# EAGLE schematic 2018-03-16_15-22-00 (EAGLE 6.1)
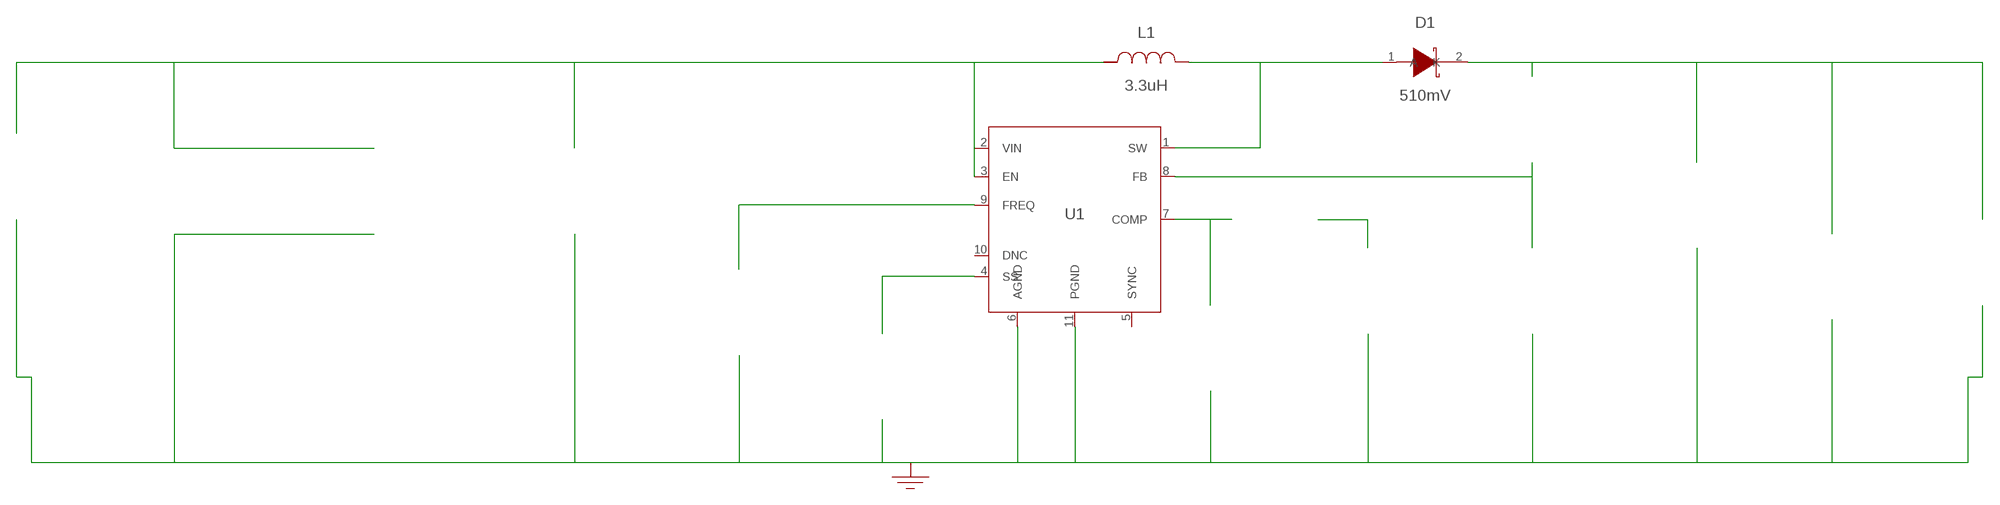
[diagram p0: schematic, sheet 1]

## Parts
CCOMP  100nF  08053C104JAZ2A08053C104JAZ2A  [0805]  (not placed on a sheet)
CCOMP2  10nF  GCM2195C1H103JA16DGCM2195C1H103JA16D  [0805]  (not placed on a sheet)
CIN  10uF  GRM219R61A106KE44DGRM219R61A106KE44D  [0805]  (not placed on a sheet)
CIN_2  10uF  GRM219R61A106KE44DGRM219R61A106KE44D  [0805]  (not placed on a sheet)
CIN_3  10uF  GRM219R61A106KE44DGRM219R61A106KE44D  [0805]  (not placed on a sheet)
CINX  100nF  CC0805KRX7R8BB104CC0805KRX7R8BB104  [0805]  (not placed on a sheet)
COUT  22uF  GRM32ER61C226ME20LGRM32ER61C226ME20L  [1210]  (not placed on a sheet)
COUTX  1uF  EMK107B7105KA-TEMK107B7105KA-T  [0603]  (not placed on a sheet)
CSS  22nF  GRM033R60J223KE01DGRM033R60J223KE01D  [0201]  (not placed on a sheet)
D1  510mV  MBRD835LT4GMBRD835LT4G  [DPAK]
GND  WB_GND  WB_GNDWB_GND  [WB_GND]
IOUT  WB_CURRENT_LOAD  WB_CURRENT_LOADWB_CURRENT_LOAD  [WB_CURRENT_LOAD]  (not placed on a sheet)
L1  3.3uH  XAL5030-332MEBXAL5030-332MEB  [XAL5030]
RCOMP  953  CRCW0402953RFKEDCRCW0402953RFKED  [0402]  (not placed on a sheet)
RFBB  10k  RR1220P-103-DRR1220P-103-D  [0805]  (not placed on a sheet)
RFBT  86.6k  CRCW040286K6FKEDCRCW040286K6FKED  [0402]  (not placed on a sheet)
RT  60.4k  CRCW040260K4FKEDCRCW040260K4FKED  [0402]  (not placed on a sheet)
U1  TPS55340RTER  TPS55340RTERTPS55340RTER  [S-PWQFN-N16]
VIN  WB_BATTERY  WB_BATTERYWB_BATTERY  [WB_BATTERY]  (not placed on a sheet)

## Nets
0: Ccomp2.1@1 Ccomp.2@2 Cin.2@2 Cin_2.2@2 Cin_3.2@2 Cinx.2@2 Cout.2@2 Coutx.2@2 Css.2@2 GND.1 Iout.-@2 Rfbb.2@2 Rt.2@2 U1.6(AGND) U1.11(PGND) U1.12(PGND) U1.13(PGND) U1.17(ETPAD) Vin.-@2
1: Cin.1@1 Cin_2.1@1 Cin_3.1@1 Cinx.1@1 L1.2 U1.2(VIN) U1.3(EN) Vin.+@1
2: Rt.1@1 U1.9(FREQ)
3: Css.1@1 U1.4(SS)
4: Ccomp2.2@2 Rcomp.2@2 U1.7(COMP)
5: D1.1(A) D1.3(A) L1.1 U1.1(SW) U1.15(SW) U1.16(SW)
6: Ccomp.1@1 Rcomp.1@1
7: Rfbb.1@1 Rfbt.2@2 U1.8(FB)
8: Cout.1@1 Coutx.1@1 D1.2(K) Iout.+@1 Rfbt.1@1
Unconnected: CCOMP2.1 CCOMP2.2 CCOMP.1 CCOMP.2 CIN.1 CIN.2 CIN_2.1 CIN_2.2 CIN_3.1 CIN_3.2 CINX.1 CINX.2 COUT.1 COUT.2 COUTX.1 COUTX.2 CSS.1 CSS.2 IOUT.1(+) IOUT.2(-) RCOMP.1 RCOMP.2 RFBB.1 RFBB.2 RFBT.1 RFBT.2 RT.1 RT.2 U1.5(SYNC) U1.10(DNC) U1.14(DNC) VIN.1(+) VIN.2(-)

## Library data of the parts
CCOMP = AcceleratedDesigns_Lib:08053C104JAZ2A; Cap: 1.0E-7; Datasheet_URL: http://catalogs.avx.com/SurfaceMount.pdf; ESR: 0.0; IRMS: 0.0; Manufacturer_Name: AVX; Manufacturer_Part_Number: 08053C104JAZ2A; VDC: 25.0; Vendor: AVX
CCOMP2 = AcceleratedDesigns_Lib:GCM2195C1H103JA16D; Cap: 1.0E-8; Datasheet_URL: http://www.murata.com/products/catalog/pdf/c03e.pdf; ESR: 0.0; IRMS: 0.0; Manufacturer_Name: MuRata; Manufacturer_Part_Number: GCM2195C1H103JA16D; VDC: 50.0; Vendor: MuRata
CIN CIN_2 CIN_3 = AcceleratedDesigns_Lib:GRM219R61A106KE44D; Cap: 1.0E-5; ESR: 0.0050; IRMS: 0.0; Manufacturer_Name: MuRata; Manufacturer_Part_Number: GRM219R61A106KE44D; VDC: 10.0; Vendor: MuRata
CINX = AcceleratedDesigns_Lib:CC0805KRX7R8BB104; Cap: 1.0E-7; ESR: 0.0; IRMS: 0.0; Manufacturer_Name: Yageo America; Manufacturer_Part_Number: CC0805KRX7R8BB104; VDC: 25.0; Vendor: Yageo America
COUT = AcceleratedDesigns_Lib:GRM32ER61C226ME20L; Cap: 2.2E-5; ESR: 0.0020; IRMS: 0.0; Manufacturer_Name: MuRata; Manufacturer_Part_Number: GRM32ER61C226ME20L; VDC: 16.0; Vendor: MuRata
COUTX = AcceleratedDesigns_Lib:EMK107B7105KA-T; Cap: 1.0E-6; ESR: 0.0; IRMS: 0.0; Manufacturer_Name: Taiyo Yuden; Manufacturer_Part_Number: EMK107B7105KA-T; VDC: 16.0; Vendor: Taiyo Yuden
CSS = AcceleratedDesigns_Lib:GRM033R60J223KE01D; Cap: 2.2E-8; ESR: 0.0; IRMS: 0.0; Manufacturer_Name: MuRata; Manufacturer_Part_Number: GRM033R60J223KE01D; VDC: 6.3; Vendor: MuRata
D1 = AcceleratedDesigns_Lib:MBRD835LT4G; Datasheet_URL: http://www.onsemi.com/pub%5Flink/Collateral/MBRD835L%2DD.PDF; Io: 8.0; Manufacturer_Name: ON Semiconductor; Manufacturer_Part_Number: MBRD835LT4G; VFatIo: 0.51; VRRM: 35.0; Vendor: ON Semiconductor
GND = AcceleratedDesigns_Lib:WB_GND; Manufacturer_Name: WB_GND; Manufacturer_Part_Number: WB_GND; PowerPortType: POWER_GROUND; Value: Value
IOUT = AcceleratedDesigns_Lib:WB_CURRENT_LOAD; Manufacturer_Name: WB_CURRENT_LOAD; Manufacturer_Part_Number: WB_CURRENT_LOAD; PowerPortType: POWER_GROUND; Value: Value
L1 = AcceleratedDesigns_Lib:XAL5030-332MEB; DCR: 0.02; IDC: 8.1; L: 3.3E-6; Manufacturer_Name: Coilcraft; Manufacturer_Part_Number: XAL5030-332MEB; Vendor: Coilcraft
RCOMP = AcceleratedDesigns_Lib:CRCW0402953RFKED; Manufacturer_Name: Vishay-Dale; Manufacturer_Part_Number: CRCW0402953RFKED; Power: 0.063; Resistance: 953.0; Tolerance: 1.0; Vendor: Vishay-Dale
RFBB = AcceleratedDesigns_Lib:RR1220P-103-D; Manufacturer_Name: Susumu Co Ltd; Manufacturer_Part_Number: RR1220P-103-D; Power: 0.1; Resistance: 10000.0; Tolerance: 0.5; Vendor: Susumu Co Ltd
RFBT = AcceleratedDesigns_Lib:CRCW040286K6FKED; Manufacturer_Name: Vishay-Dale; Manufacturer_Part_Number: CRCW040286K6FKED; Power: 0.063; Resistance: 86600.0; Tolerance: 1.0; Vendor: Vishay-Dale
RT = AcceleratedDesigns_Lib:CRCW040260K4FKED; Manufacturer_Name: Vishay-Dale; Manufacturer_Part_Number: CRCW040260K4FKED; Power: 0.063; Resistance: 60400.0; Tolerance: 1.0; Vendor: Vishay-Dale
U1 = AcceleratedDesigns_Lib:TPS55340RTER; Datasheet_URL: http://www.ti.com/product/tps55340; Frequency: 1200000.0; Imax: 5.0; Manufacturer_Name: Texas Instruments; Manufacturer_Part_Number: TPS55340RTER; Mktg_Package: HTSSOP; Package: HTSSOP; Vendor: Texas Instruments
VIN = AcceleratedDesigns_Lib:WB_BATTERY; Manufacturer_Name: WB_BATTERY; Manufacturer_Part_Number: WB_BATTERY; PowerPortType: POWER_GROUND; Value: Value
